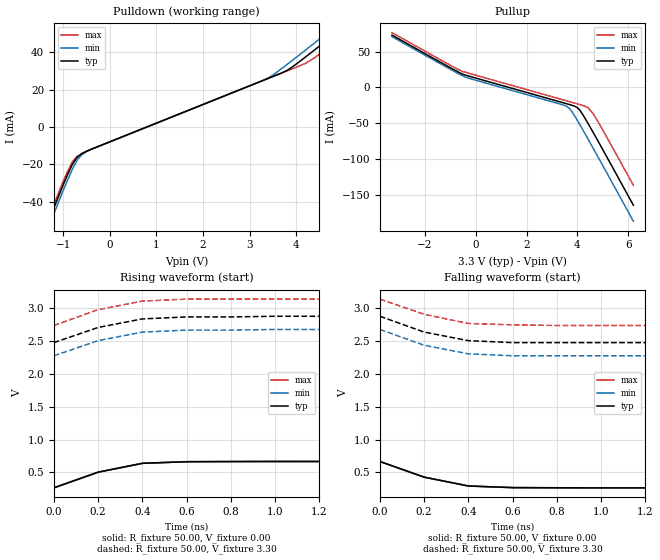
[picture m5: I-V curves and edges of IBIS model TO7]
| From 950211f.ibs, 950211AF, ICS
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|   Model TO7
[Model]   TO7
Model_type   Output
Polarity   Non-Inverting
C_comp   5.50pF   5.00pF   6.00pF
[Temperature Range]   27.00   70.00   0.00
[Voltage Range]   3.30V   3.00V   3.70V
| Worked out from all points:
|   slope of the pulldown table from 0 to 0.495 V, typ, clamps not added: 100 ohm
|   slope of the pullup table from 0 to 0.495 V, typ, clamps not added: 100 ohm
|   rising waveform, R_fixture 50.00, V_fixture 0.00: 20-80 % time 255ps typ, 256ps min, 254ps max; typ from 0.267 V to 0.667 V
|   rising waveform, R_fixture 50.00, V_fixture 3.30: 20-80 % time 269ps typ, 269ps min, 256ps max; typ from 2.47 V to 2.87 V
|   falling waveform, R_fixture 50.00, V_fixture 0.00: 20-80 % time 255ps typ, 256ps min, 254ps max; typ from 0.667 V to 0.267 V
|   falling waveform, R_fixture 50.00, V_fixture 3.30: 20-80 % time 256ps typ, 256ps min, 259ps max; typ from 2.87 V to 2.47 V
[Pulldown]
| voltage   I(typ)   I(min)   I(max)
-3.3V     -178mA     -180.9mA   -176.2mA
-1.5V     -62.15mA   -65.21mA   -60.26mA
-1V       -31.1mA    -34.13mA   -29.25mA
-800mV    -20mA      -22.63mA   -18.62mA
-600mV    -14.39mA   -14.87mA   -14.26mA
3.4V      26mA       26.19mA    26mA
3.8V      30.18mA    33.35mA    30mA
4.2V      37.43mA    41.13mA    34.02mA
4.8V      49.18mA    52.96mA    44.79mA
5V        53.13mA    56.92mA    48.71mA
5.2V      57.09mA    60.88mA    52.65mA
6.2V      76.96mA    80.76mA    72.49mA
[Pullup]
| voltage   I(typ)   I(min)   I(max)
-3.3V     72.92mA    70.75mA    76.41mA
-1V       27.37mA    25.22mA    30.84mA
-500mV    18.18mA    15.78mA    22.02mA
3.6V      -23mA      -26.87mA   -19mA
3.7V      -24mA      -29.83mA   -20mA
3.8V      -25.07mA   -34.63mA   -21mA
4V        -28.26mA   -46.13mA   -23mA
4.1V      -32mA      -52.21mA   -24mA
4.4V      -49.14mA   -70.89mA   -27.83mA
4.6V      -61.54mA   -83.55mA   -35.54mA
5V        -86.87mA   -109.1mA   -59.64mA
6.2V      -164.1mA   -186.5mA   -136.4mA
[Ramp]
| variable   typ   min   max
dV/dt_r   240.00m/187.94p   240.00m/189.70p   240.00m/186.05p
dV/dt_f   240.00m/200.00p   240.00m/200.00p   240.00m/200.00p
[Rising Waveform]
R_fixture = 50.00
V_fixture = 0.00
V_fixture_min = 0.00
V_fixture_max = 0.00
| time   V(typ)   V(min)   V(max)
0s        266.7mV    266.7mV    266.7mV
200ps     504.4mV    503.8mV    505.1mV
400ps     639.1mV    638.1mV    640mV
600ps     663.5mV    663mV      663.9mV
1ns       667mV      667.1mV    667mV
10ns      666.7mV    666.7mV    666.7mV
[Rising Waveform]
R_fixture = 50.00
V_fixture = 3.30
V_fixture_min = 3.00
V_fixture_max = 3.70
| time   V(typ)   V(min)   V(max)
0s        2.47V      2.27V      2.73V
200ps     2.7V       2.5V       2.97V
400ps     2.83V      2.63V      3.1V
600ps     2.86V      2.66V      3.13V
800ps     2.86V      2.66V      3.13V
1ns       2.87V      2.67V      3.13V
10ns      2.87V      2.67V      3.13V
[Falling Waveform]
R_fixture = 50.00
V_fixture = 0.00
V_fixture_min = 0.00
V_fixture_max = 0.00
| time   V(typ)   V(min)   V(max)
0s        666.7mV    666.7mV    666.7mV
200ps     428.6mV    429.3mV    427.9mV
400ps     294.4mV    295.5mV    293.5mV
600ps     269.9mV    270.4mV    269.5mV
1ns       266.3mV    266.2mV    266.3mV
10ns      266.7mV    266.7mV    266.7mV
[Falling Waveform]
R_fixture = 50.00
V_fixture = 3.30
V_fixture_min = 3.00
V_fixture_max = 3.70
| time   V(typ)   V(min)   V(max)
0s        2.87V      2.67V      3.13V
200ps     2.63V      2.43V      2.9V
400ps     2.5V       2.3V       2.76V
600ps     2.47V      2.27V      2.74V
800ps     2.47V      2.27V      2.73V
10ns      2.47V      2.27V      2.73V
